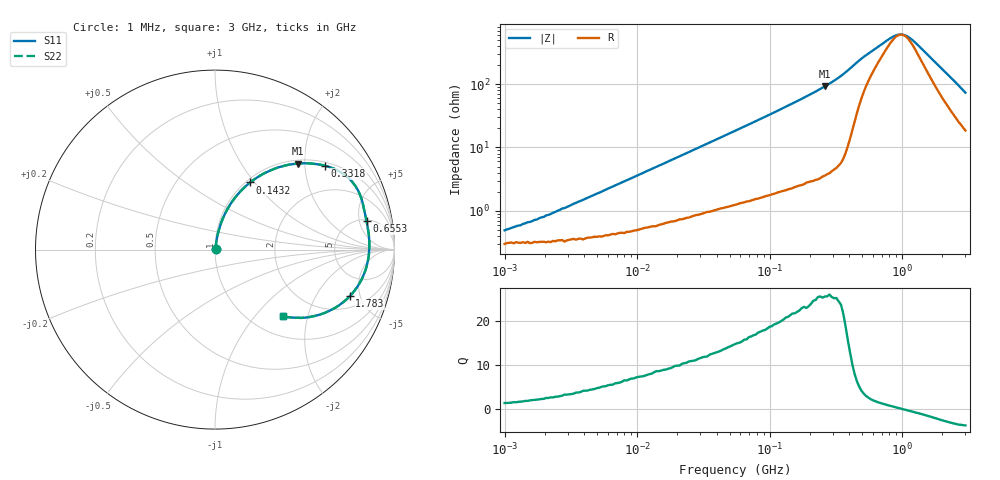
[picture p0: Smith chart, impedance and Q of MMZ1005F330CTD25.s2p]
! S-Parameter Data Generated by TDK Corporation
! Copyright(C) 2025 TDK Corporation.
! All Rights Reserved.
! TDK P/N: MMZ1005F330CTD25 (Chip Bead)
! Property: |Z|=33ohm at 100MHz
! Size(LxWxT): 1x0.5x0.5mm
! Model Type: s2p (Touchstone File Format Version 1.0)
! Frequency: DC=Yes Start=1MHz Stop=3000MHz 202points Log-sweep
! Model Generated on Feb. 6, 2025
! Terms and conditions regarding TDK Simulation Models:
! 1)This simulation model is being provided solely for informational
!  purposes. Please refer to the specifications of the products in
!  terms of detailed characteristics of such products.
! 2)In no event shall TDK Corporation of any of its subsidiaries be
!  liable for any loss or damage arising, directly or indirectly,
!  from any information contained in this simulation model, including,
!  but not limited to loss or damages arising from any inaccuracies,
!  omissions or errors in connection with such information.
! 3)Any and all copyrights on this simulation model are owned by
!  TDK Corporation.  Duplication or redistribution of this simulation
!  model without prior written permission from TDK Corporation
!  is prohibited.
! 4)This simulation model is subject to any modification or change
!  without any prior notice.
! 5)Neither TDK Corporation nor any of its subsidiaries shall make any
!  warranty, express or implied, including but not limited to the
!  correctness, implied warranties of merchantability and fitness for
!  a particular purpose with respect to this simulation models.
! 6)The use of this simulation model shall be deemed to have consented
!  to the terms and conditions hereof.
! Port Assignments:
!  1 ---@@@--- 2
! Applicable Conditions:
!  Temperature = 25 degC
!  DC Bias Current = 0 A
!  Small Signal Operation
# Hz S MA R 50
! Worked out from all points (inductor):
!   201 points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, 1 MHz to 3 GHz, reference 50 ohm
!   read as one part in series: L = 58.9 nH near 2.832 MHz
!   highest Q = 25.7 at 261 MHz (marker M1), where L = 56.3 nH
!   self-resonance near 988.5 MHz
!   S11 on the Smith chart (normalised r, x): 1 MHz: 1.01, +0.01; 143.2 MHz: 1.04, +0.95; 331.8 MHz: 1.10, +2.54; 655.3 MHz: 5.33, +6.44; 1.783 GHz: 2.84, -4.00; 3 GHz: 1.37, -1.42
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1000000  0.004885 52.3  0.997 -0.2  0.997 -0.2  0.004885 52.3
1974946  0.007952 65.7  0.9968 -0.4  0.9968 -0.4  0.007952 65.7
3900413  0.0148 75.5  0.9964 -0.8  0.9964 -0.8  0.0148 75.5
1.461624e7  0.05127 80.4  0.9928 -2.9  0.9928 -2.9  0.05127 80.4
3.00453e7  0.1012 79.3  0.9862 -5.8  0.9862 -5.8  0.1012 79.3
5.477226e7  0.178 75.9  0.9721 -10.2  0.9721 -10.2  0.178 75.9
9.593103e7  0.2979 69.6  0.9385 -17.3  0.9385 -17.3  0.2979 69.6
1.431579e8  0.4225 62.4  0.8869 -25.0  0.8869 -25.0  0.4225 62.4
2.136344e8  0.5796 52.3  0.7918 -35.4  0.7918 -35.4  0.5796 52.3
2.609752e8  0.6659 46.1  0.7206 -41.7  0.7206 -41.7  0.6659 46.1
3.318279e8  0.7709 37.3  0.6064 -50.4  0.6064 -50.4  0.7709 37.3
3.894533e8  0.8328 30.1  0.503 -56.2  0.503 -56.2  0.8328 30.1
4.570858e8  0.8625 22.4  0.3863 -58.4  0.3863 -58.4  0.8625 22.4
6.553423e8  0.8593 10.6  0.2216 -45.5  0.2216 -45.5  0.8593 10.6
8.005644e8  0.8612 5.5  0.165 -30.1  0.165 -30.1  0.8612 5.5
9.395906e8  0.8602 1.4  0.1416 -8.4  0.1416 -8.4  0.8602 1.4
1.059487e9  0.8577 -1.9  0.1455 11.2  0.1455 11.2  0.8577 -1.9
1.194682e9  0.8518 -5.3  0.1706 27.2  0.1706 27.2  0.8518 -5.3
1.402151e9  0.8382 -10.3  0.2305 40.5  0.2305 40.5  0.8382 -10.3
1.782824e9  0.7943 -19.1  0.3607 46.2  0.3607 46.2  0.7943 -19.1
2.359433e9  0.6858 -31.9  0.5535 41.0  0.5535 41.0  0.6858 -31.9
3e9  0.5315 -44.4  0.7234 31.0  0.7234 31.0  0.5315 -44.4
